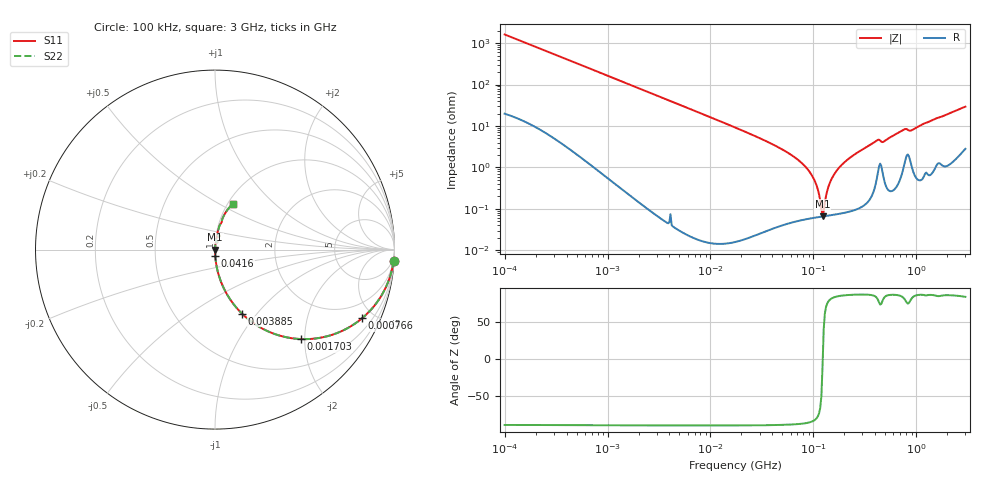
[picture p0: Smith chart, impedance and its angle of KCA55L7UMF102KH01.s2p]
!Murata Part Number: KCA55L7UMF102KH01
!These Parameters are Measured in Series Mode Connection
!Data Generated on Jan 08, 2026
!  o--ll--o
!Port1  Port2
!  o------o
!Operation Temp=25[degC], DC Bias Voltage=0[V]
!Freq. Start=100[kHz] Stop=3[GHz] 401[Steps]
# Hz S RI R 50
!Freq.(Hz) S11(Real) S11(Imag) S21(Real) S21(Imag) S12(Real) S12(Imag) S22(Real) S22(Imag)
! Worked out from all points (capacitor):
!   401 points, 100 kHz to 3 GHz, reference 50 ohm
!   read as one part in series: C = 985 pF near 105.3 kHz
!   lowest |Z| = 66.7 mohm at 122.8 MHz (marker M1)
!   series resonance near 123.3 MHz, so ESL is about 1.7 nH
!   S11 on the Smith chart (normalised r, x): 100 kHz: 1, -32; 766 kHz: 1.02, -4.27; 1.703 MHz: 1.00, -1.92; 3.885 MHz: 1.00, -0.84; 41.6 MHz: 1.00, -0.07; 3 GHz: 1.06, +0.58
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100000  0.9954 -0.0618  0.0046 0.0618  0.0046 0.0618  0.9954 -0.0618
562235  0.8927 -0.3066  0.1073 0.3066  0.1073 0.3066  0.8927 -0.3066
766005  0.8189 -0.383  0.1811 0.383  0.1811 0.383  0.8189 -0.383
1702975  0.4798 -0.4986  0.5202 0.4986  0.5202 0.4986  0.4798 -0.4986
3161081  0.2113 -0.4076  0.7887 0.4076  0.7887 0.4076  0.2113 -0.4076
3884884  0.1505 -0.357  0.8495 0.357  0.8495 0.357  0.1505 -0.357
1.77727e7  0.00819 -0.0892  0.9918 0.0892  0.9918 0.0892  0.00819 -0.0892
4.160216e7  0.00154 -0.0346  0.9985 0.0346  0.9985 0.0346  0.00154 -0.0346
7.147675e7  0.00074 -0.015  0.9993 0.015  0.9993 0.015  0.00074 -0.015
9.738194e7  0.000639 -0.00624  0.9994 0.00624  0.9994 0.00624  0.000639 -0.00624
1.079567e8  0.000639 -0.00349  0.9994 0.00349  0.9994 0.00349  0.000639 -0.00349
1.196798e8  0.000653 -0.000781  0.9993 0.000781  0.9993 0.000781  0.000653 -0.000781
1.228043e8  0.000659 -0.000105  0.9993 0.000105  0.9993 0.000105  0.000659 -0.000105
1.293002e8  0.000673 0.00125  0.9993 -0.00125  0.9993 -0.00125  0.000673 0.00125
1.361397e8  0.000691 0.0026  0.9993 -0.0026  0.9993 -0.0026  0.000691 0.0026
1.470833e8  0.000727 0.00465  0.9993 -0.00465  0.9993 -0.00465  0.000727 0.00465
1.854806e8  0.000898 0.011  0.9991 -0.011  0.9991 -0.011  0.000898 0.011
4.018672e8  0.00563 0.0421  0.9944 -0.0421  0.9944 -0.0421  0.00563 0.0421
5.475153e8  0.00538 0.0514  0.9946 -0.0514  0.9946 -0.0514  0.00538 0.0514
7.459503e8  0.0152 0.078  0.9848 -0.078  0.9848 -0.078  0.0152 0.078
8.934279e8  0.0171 0.075  0.9829 -0.075  0.9829 -0.075  0.0171 0.075
3e9  0.0996 0.255  0.9004 -0.255  0.9004 -0.255  0.0996 0.255
